FUNCTION_BLOCK Axis_PTP_1 IMPLEMENTS ITF_Axis_Ex, ITF_Axis_Ex
VAR_INPUT
	DrvIn:ST_DrvIn;
	PARA:ST_AxisPara;
END_VAR

VAR_OUTPUT
	Status:ST_AxisStatus;	
END_VAR
VAR
	REF: AXIS_REF;
	mcPower: mc_Power;
END_VAR

;

METHOD M_Cyclic : BOOL
// 2018.03.27 By Lizzy Chen
// Method and Action could be inherited, while code in root of FB can't be inherited.
// That's why create this Method.
VAR_INPUT
END_VAR
;
REF.ReadStatus();
Status.Axis_Ready:=REF.Status.ControlLoopClosed;
Status.Axis_Err:=REF.Status.Error;
Status.Axis_IsPTP:=REF.Status.PTPmode;
Status.Current_Pos:=REF.NcToPlc.ActPos;
END_METHOD

METHOD M_Home : BOOL
VAR_INPUT
	Execute:BOOL;
END_VAR
VAR_STAT
	mcHome:Tc2_MC2.MC_Home;
END_VAR
mcHome(
	Axis:= REF, 
	Execute:= Execute, 
	Position:= PARA.RefPos,
	bCalibrationCam:= DrvIn.HomeSensor);
END_METHOD

{warning 'add method implementation'}
METHOD M_MoveVel : BOOL
VAR_INPUT
	Execute	: BOOL;
END_VAR
VAR_STAT
	mcMoveVel: Tc2_MC2.MC_MoveVelocity;
END_VAR
mcMoveVel(
	Axis:= REF, 
	Execute:= Execute, 
	Velocity:= PARA.MoveVelo  );
END_METHOD

{warning 'add method implementation'}
METHOD M_PowerOff : BOOL
VAR_INPUT

END_VAR

VAR

END_VAR
mcPower(
	Axis:= REF, 
	Enable:=FALSE , 
	Enable_Positive:=TRUE , 
	Enable_Negative:=TRUE , 
	Override:=PARA.rOverride  );
END_METHOD

{warning 'add method implementation'}
METHOD M_PowerOn : BOOL
VAR_INPUT

END_VAR

VAR

END_VAR
mcPower(
	Axis:= REF, 
	Enable:=TRUE , 
	Enable_Positive:=TRUE , 
	Enable_Negative:=TRUE , 
	Override:=PARA.rOverride  );
END_METHOD

METHOD M_Reset : BOOL
VAR_INPUT
	Execute:BOOL;
END_VAR
VAR_STAT
	mcReset:Tc2_MC2.MC_Reset;
END_VAR
mcReset(
	Axis:=REF , 
	Execute:=EXECUTE);
END_METHOD

{warning 'add method implementation'}
METHOD M_Stop : BOOL
VAR_INPUT
	Execute	: BOOL;
END_VAR
END_METHOD

{warning 'add property implementation'}
PROPERTY P_Status : ST_AxisStatus
GET
END_GET
SET

P_Status.Axis_Ready:=REF.Status.ControlLoopClosed;
P_Status.Axis_IsPTP:=REF.Status.PTPmode;
END_SET
END_PROPERTY

END_FUNCTION_BLOCK
